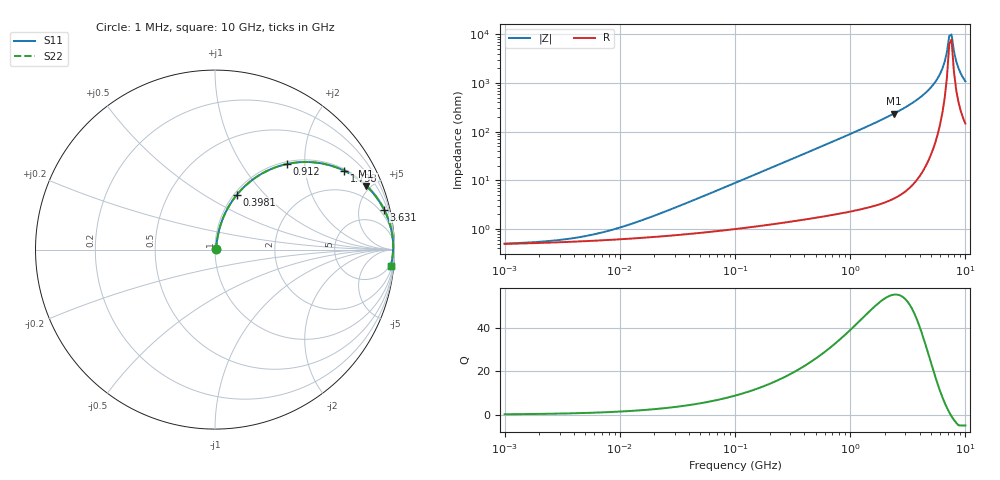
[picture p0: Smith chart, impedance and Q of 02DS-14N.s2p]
# MHz S MA R 50
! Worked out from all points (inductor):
!   201 points, 1 MHz to 10 GHz, reference 50 ohm
!   read as one part in series: L = 14 nH near 25.12 MHz
!   highest Q = 55.4 at 2.399 GHz (marker M1), where L = 15.6 nH
!   self-resonance near 7.244 GHz
!   S11 on the Smith chart (normalised r, x): 1 MHz: 1.01, +0.00; 398.1 MHz: 1.03, +0.70; 912 MHz: 1.04, +1.63; 1.738 GHz: 1.06, +3.23; 3.631 GHz: 1.18, +8.39; 10 GHz: 4, -21
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1  0.005013 10.0  0.9951 -0.1  0.9951 -0.1  0.005013 10.0
4.7863  0.006987 36.6  0.9944 -0.2  0.9944 -0.2  0.006987 36.6
9.54993  0.01034 53.4  0.9939 -0.5  0.9939 -0.5  0.01034 53.4
21.8776  0.02034 68.9  0.9928 -1.1  0.9928 -1.1  0.02034 68.9
104.713  0.09138 78.5  0.9859 -5.2  0.9859 -5.2  0.09138 78.5
398.107  0.3271 68.4  0.9305 -19.1  0.9305 -19.1  0.3271 68.4
478.63  0.3842 65.2  0.9081 -22.6  0.9081 -22.6  0.3842 65.2
912.011  0.6235 49.9  0.7652 -38.6  0.7652 -38.6  0.6235 49.9
1737.8  0.8433 31.4  0.5214 -57.5  0.5214 -57.5  0.8433 31.4
2187.76  0.8972 25.2  0.4257 -63.8  0.4257 -63.8  0.8972 25.2
2398.83  0.9146 22.8  0.3882 -66.1  0.3882 -66.1  0.9146 22.8
3630.78  0.9681 13.3  0.2307 -75.4  0.2307 -75.4  0.9681 13.3
4786.3  0.9857 7.9  0.137 -80.1  0.137 -80.1  0.9857 7.9
5754.4  0.9914 4.5  0.07857 -81.4  0.07857 -81.4  0.9914 4.5
6606.93  0.9929 2.1  0.03639 -77.7  0.03639 -77.7  0.9929 2.1
6918.31  0.9929 1.2  0.02284 -71.2  0.02284 -71.2  0.9929 1.2
7244.36  0.9926 0.4  0.01071 -46.2  0.01071 -46.2  0.9926 0.4
7585.78  0.9921 -0.4  0.009992 37.7  0.009992 37.7  0.9921 -0.4
7943.28  0.9914 -1.2  0.0218 66.1  0.0218 66.1  0.9914 -1.2
8317.64  0.9903 -2.0  0.03524 73.1  0.03524 73.1  0.9903 -2.0
9120.11  0.9875 -3.6  0.06293 76.8  0.06293 76.8  0.9875 -3.6
10000  0.9835 -5.2  0.09109 77.0  0.09109 77.0  0.9835 -5.2
